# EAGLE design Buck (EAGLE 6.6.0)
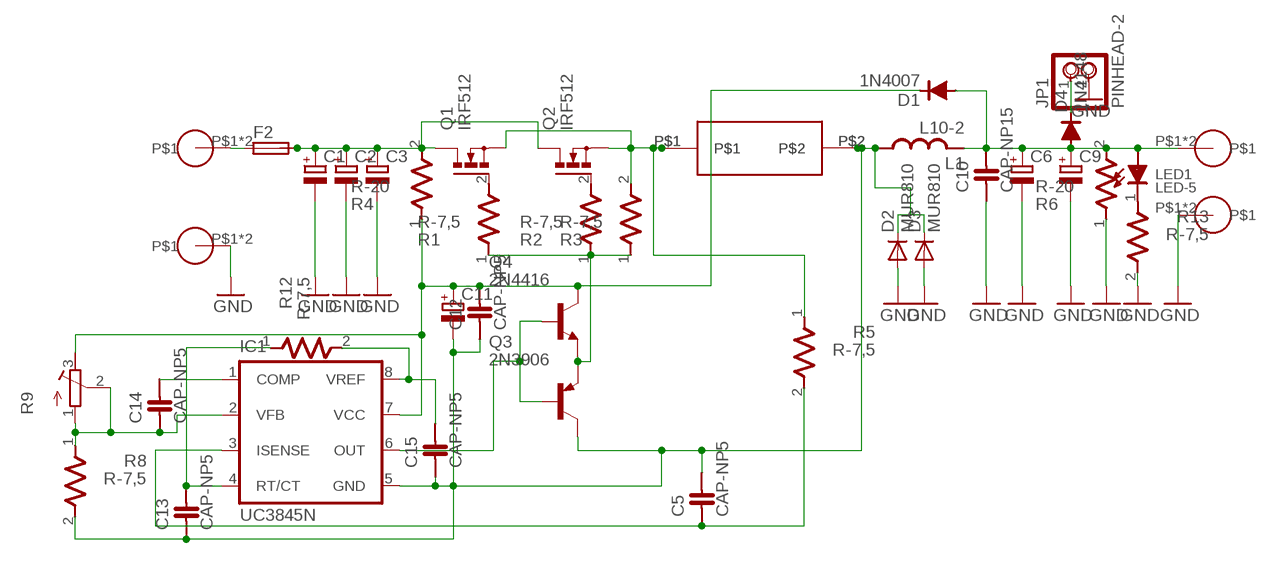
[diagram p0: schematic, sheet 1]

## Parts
C1  CPOL-EUE7.5-18  [E7,5-18]
C2  CPOL-EUE7.5-18  [E7,5-18]
C3  CPOL-EUE7.5-18  [E7,5-18]
C5  CAP-NP5  [CAP-NP5]
C6  CPOL-EUE7.5-18  [E7,5-18]
C9  CPOL-EUE7.5-18  [E7,5-18]
C10  CAP-NP15  [CAP-NP-15]
C11  CPOL-EUE5-8.5  [E5-8,5]
C12  CAP-NP5  [CAP-NP5]
C13  CAP-NP5  [CAP-NP5]
C14  CAP-NP5  [CAP-NP5]
C15  CAP-NP5  [CAP-NP5]
D1  1N4007  [1N4007]
D2  MUR810  [TO220ACS]
D3  MUR810  [TO220ACS]
D4  1N4148  [D-7,5]
F2  LITTLEFUSE  [LITTLEFUSE]
IC1  UC3845N  [DIL08]
JP1  PINHEAD-2  [PINHEAD-2]
L1  L10-2  [L10-2]
LED1  LED-5  [LED5]
Q1  IRF512  [TO220BV]
Q2  IRF512  [TO220BV]
Q3  2N3906  [TO92]
Q4  2N4416  [TO92]
R1  R-7,5  [R-7,5]
R2  R-7,5  [R-7,5]
R3  R-7,5  [R-7,5]
R4  R-20  [R-20]
R5  R-7,5  [R-7,5]
R6  R-20  [R-20]
R8  R-7,5  [R-7,5]
R9  R-TRIMM64W  [RTRIM64W]
R12  R-7,5  [R-7,5]
R13  R-7,5  [R-7,5]
U$1  PIN5MM  [PIN5MM]
U$2  PIN5MM  [PIN5MM]
U$3  SHUNT-0.01R  [SHUNT-0.01R]
U$4  PIN5MM  [PIN5MM]
U$5  PIN5MM  [PIN5MM]
U$6  SHUNT-0.01R  [SHUNT-0.01R]

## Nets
GND: C1.- C2.- C3.- C6.- C9.- C10.1 D2.A D3.A JP1.2 R6.1 R13.2 U$1.P$1 U$1.P$2 U$5.P$1 U$5.P$2
N$1: F2.1 U$2.P$1 U$2.P$2
N$2: C1.+ C2.+ C3.+ F2.2 Q1.D Q2.D R4.2
N$3: Q1.G R1.2
N$4: Q2.G R2.2
N$5: LED1.K R13.1
N$6: D4.C JP1.1
N$7: IC1.6(OUT) Q3.2(B) Q4.2(B)
N$8: Q3.3(E) Q4.3(E) R1.1 R2.1 R3.1
N$9: C5.1 IC1.3(ISENSE) R5.2
N$10: C11.+ C12.2 D1.K IC1.7(VCC) Q4.1(C) R4.1 R9.3(E)
N$11: C6.+ C9.+ C10.2 D1.A D4.A L1.P$3 L1.P$4 LED1.A R6.2 U$4.P$1 U$4.P$2
N$12: C14.2 IC1.1(COMP)
N$13: C5.2 C11.- C12.1 C13.1 C15.1 D2.C D3.C IC1.5(GND) L1.P$1 L1.P$2 Q3.1(C) R8.2 U$3.P$2 U$6.P$2
N$14: Q1.S Q2.S R3.2 R5.1 U$3.P$1 U$6.P$1
N$15: C14.1 IC1.2(VFB) R8.1 R9.1(A) R9.2(S)
N$18: C15.2 IC1.8(VREF) R12.2
N$19: C13.2 IC1.4(RT/CT) R12.1

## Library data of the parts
C1-C3 C6 C9 C11 = LBR inverter true sine:CPOL-EU: POLARIZED CAPACITOR, European symbol
C5 C12-C15 = chuong:CAP-NP5
C10 = chuong:CAP-NP15
D1 = chuong:1N4007
D2 D3 = lbr:MUR810: DIODE
D4 = chuong:1N4148
F2 = LBR inverter true sine:LITTLEFUSE: LITTLEFUSE; OC_FARNELL: unknown; OC_NEWARK: unknown
IC1 = v-reg:UC384*: SMPS Controller Source: http://www.fairchildsemi.com/ds/UC/UC3843.pdf
JP1 = chuong:PINHEAD-2
L1 = lbr:L10-2
LED1 = chuong:LED-5
Q1 Q2 = LBR inverter true sine:IRF512: N-CHANNEL MOS FET
Q3 = lbr:2N3906: PNP Transistor
Q4 = lbr:2N4416: NPN Transistor
R1-R3 R5 R8 R12 R13 = chuong:R-7,5
R4 R6 = chuong:R-20
R9 = chuong:R-TRIMM: Trimm resistor
U$1 U$2 U$4 U$5 = LBR inverter true sine:PIN5MM
U$3 U$6 = Shunt 0.01R:SHUNT-0.01R

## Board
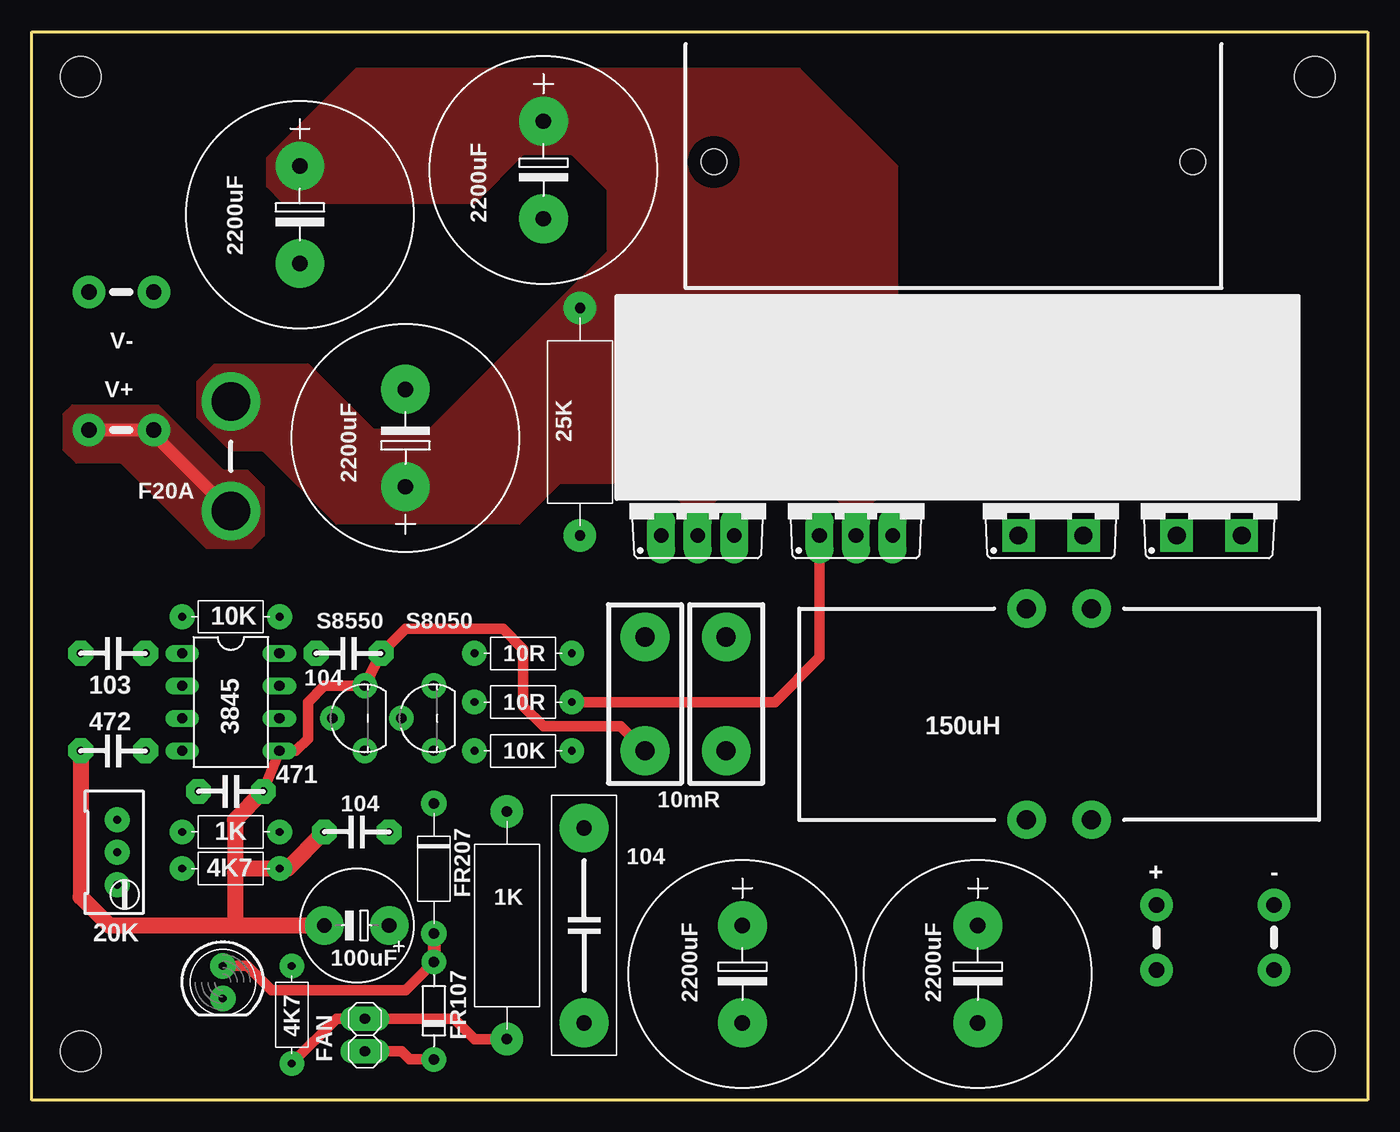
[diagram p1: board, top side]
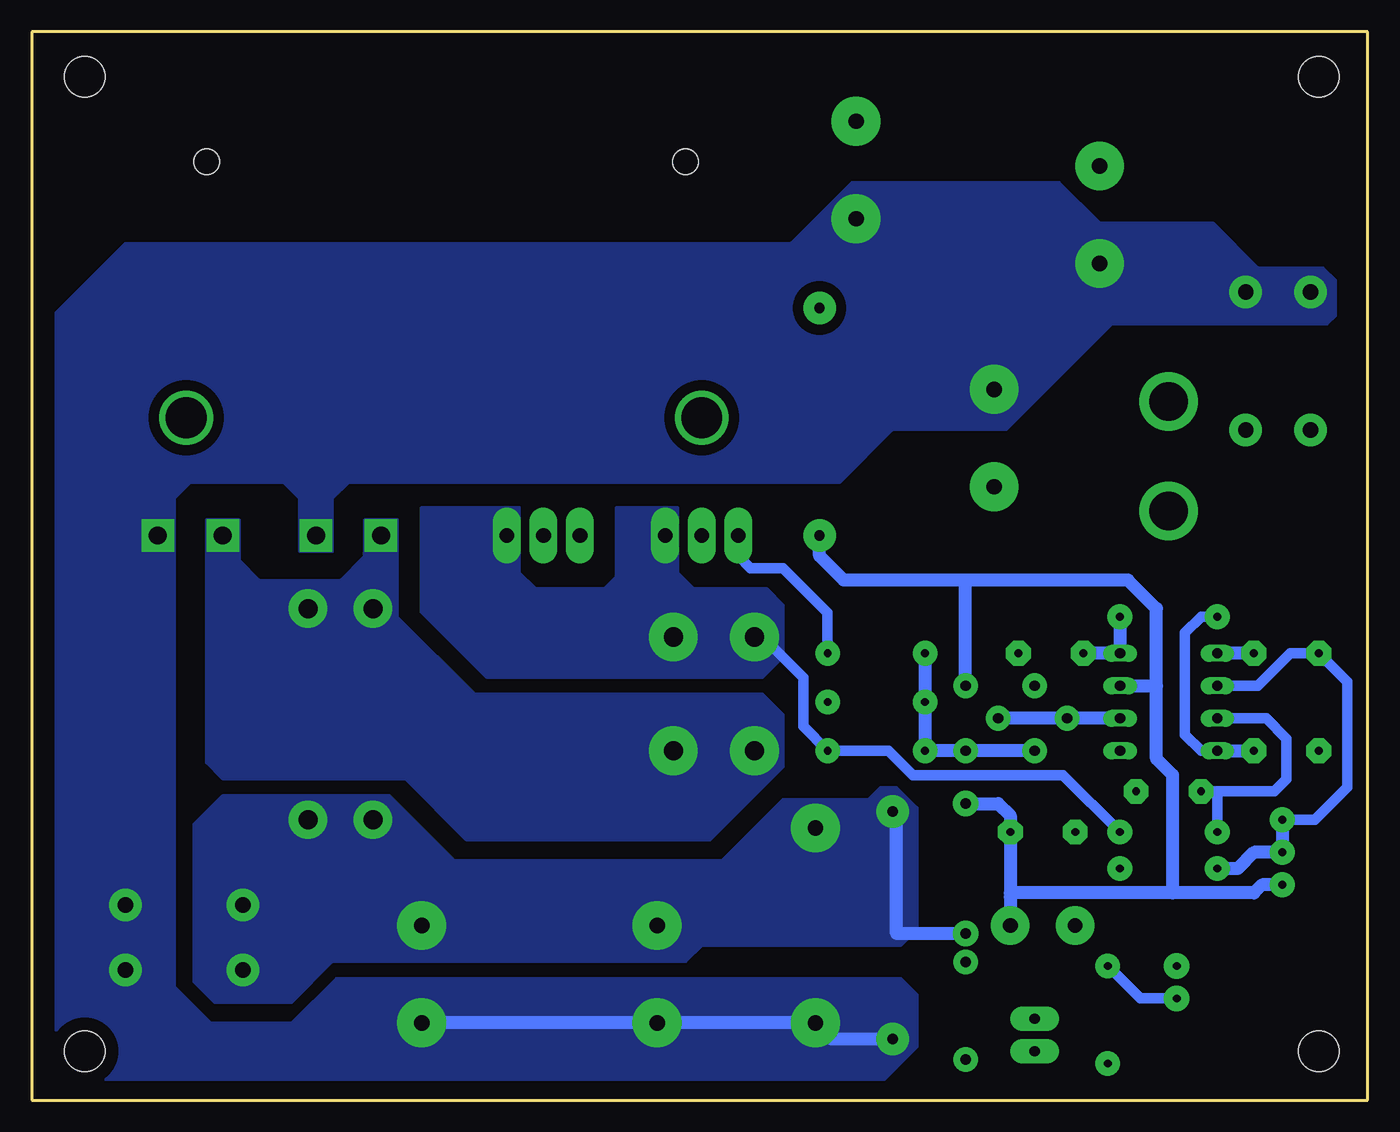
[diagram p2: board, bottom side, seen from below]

Size 104.46 x 83.5 mm. Coordinates in mm from the lower left corner, seen from the top.
Outline: 0,83.5 104.46,83.5 104.46,0 0,0 0,83.5
Copper layers (1*16): Top 0.035mm / dielectric 1.5mm / Bottom 0.035mm
Design rules "default": minimum track width 10mil, minimum drill 24mil, track to track 8mil, track to pad 8mil, pad to pad 8mil, via to via 8mil, smd to smd 8mil, copper to edge 40mil, drill to drill 8mil, minimum pad ring 10mil, minimum via ring 8mil, stop-mask expansion 4mil, vias tented up to drill 0mil, thermal gap 10mil
Holes 2 mm at 90.8,73.34 53.34,73.34
Holes 3.2 mm at 3.81,3.81 100.33,3.81 3.81,80.01 100.33,80.01

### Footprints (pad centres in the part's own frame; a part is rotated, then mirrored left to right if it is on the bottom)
E7,5-18 = drill 1.2 pad 3.81: + -3.81,0; - 3.81,0
CAP-NP5 = drill 0.61 pad 1.93 octagon: 1 -3.81,0; 2 1.27,0
CAP-NP-15 = drill 1.2 pad 3.81: 1 -13.97,0; 2 1.27,0
E5-8,5 = drill 1.15 pad 3: + -2.54,0; - 2.54,0
1N4007 = drill 0.8 pad 2: A 5.08,0; K -5.08,0
TO220ACS = drill 1.4 pad 2.54 square: A 2.54,-2.54; C -2.54,-2.54
D-7,5 = drill 0.8 pad 1.93: A 3.81,0; C -3.81,0
LITTLEFUSE = drill 3 pad 4.572: 1 -5.08,0; 2 3.493,0
DIL08 = drill 0.813 long: 1 -3.81,-3.81; 2 -1.27,-3.81; 3 1.27,-3.81; 4 3.81,-3.81; 5 3.81,3.81; 6 1.27,3.81; 7 -1.27,3.81; 8 -3.81,3.81
PINHEAD-2 = drill 0.813 pad 1.93 long: 1 -1.27,0; 2 1.27,0
L10-2 = drill 1.5 pad 3: P$1 -8.89,2.54; P$2 -8.89,-2.54; P$3 7.62,-2.54; P$4 7.62,2.54
LED5 = drill 0.61 pad 2: A -1.27,0; K 1.27,0
TO220BV = drill 1.15 pad 2.184 long: D 0,-2.54; G -2.857,-2.54; S 2.857,-2.54
TO92 = drill 0.813 pad 1.93: 1 2.54,0; 2 0,2.54; 3 -2.54,0
R-7,5 = drill 0.61 pad 1.93: 1 -3.81,0; 2 3.81,0
R-20 = drill 0.813 pad 2.54: 1 -8.89,0; 2 8.89,0
RTRIM64W = drill 0.61 pad 1.93: 1 0,-2.54; 2 0,0; 3 0,2.54
PIN5MM = drill 1.2 pad 2.54: P$1 -2.54,0; P$2 2.54,0
SHUNT-0.01R = drill 1.5 pad 3.81: P$1 -2.54,-1.27; P$2 6.35,-1.27

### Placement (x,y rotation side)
C1  20.95,69.22 270 top
C2  40.01,72.71 270 top
C3  29.21,51.75 90 top
C5  16.83,24.13 0 top
C6  73.98,9.84 270 top
C9  55.56,9.84 270 top
C10  43.18,20 90 top
C11  25.4,13.65 180 top
C12  26.67,20.96 0 top
C13  7.62,27.3 0 top
C14  7.62,34.92 0 top
C15  23.5,34.92 180 top
D1  31.43,18.1 270 top
D2  79.69,46.67 0 top
D3  92.08,46.67 0 top
D4  31.43,6.99 90 top
F2  15.56,51.12 90 top
IC1  15.56,31.12 270 top
JP1  26.04,5.08 90 top
L1  80.33,29.53 270 top
LED1  14.92,9.21 270 top
Q1  64.45,46.67 0 top
Q2  52.07,46.67 0 top
Q3  26.04,29.85 90 top
Q4  31.43,29.85 90 top
R1  38.42,31.12 0 top
R2  38.42,34.92 0 top
R3  38.42,27.3 0 top
R4  42.86,53.02 90 top
R5  15.56,20.96 180 top
R6  37.15,13.65 90 top
R8  15.56,18.1 0 top
R9  6.67,19.37 180 top
R12  15.56,37.78 0 top
R13  20.32,6.67 270 top
U$1  6.99,63.18 0 top
U$2  6.99,52.39 0 top
U$3  55.56,33.65 270 top
U$4  87.95,12.7 270 top
U$5  97.16,12.7 90 top
U$6  49.21,33.65 270 top

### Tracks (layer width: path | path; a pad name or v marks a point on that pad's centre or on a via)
GND
  Top 0.813: R6.1 34.61,4.76 33.02,6.35 JP1.2 23.81,6.35 R13.2
  Bottom 1.016: R6.1 41.91,4.76 C10.1 C9.- C6.-
  pour Bottom (isolate 0.813, no thermals): 97.16,66.99 45.09,66.99 40.32,71.76 24.13,71.76 20.95,68.58 12.06,68.58 8.57,65.09 3.49,65.09 2.54,64.14 2.54,61.28 3.18,60.64 20,60.64 28.26,52.39 37.15,52.39 41.27,48.26 79.69,48.26 80.96,46.99 80.96,42.86 83.5,42.86 83.5,46.99 84.77,48.26 92.08,48.26 93.34,46.99 93.34,8.89 90.49,6.03 84.14,6.03 80.64,9.52 36.51,9.52 35.24,8.25 35.24,4.13 37.78,1.59 98.74,1.59 102.55,5.4 102.55,61.59
N$1
  Top 1.016: U$2.P$1 U$2.P$2 9.52,52.07 F2.1 15.88,45.72
  pour Top (no thermals): 3.18,54.29 9.84,54.29 14.92,49.21 16.83,49.21 18.1,47.94 18.1,44.13 17.14,43.18 13.65,43.18 6.99,49.85 3.49,49.85 2.54,50.8 2.54,53.66
N$2  (via drill 3.2)
  other vias: 52.07,53.34
  pour Top (isolate 1.016, no thermals): 25.4,80.65 60.01,80.65 67.63,73.03 67.63,48.26 65.41,46.04 65.41,42.86 63.5,42.86 63.5,46.04 61.28,48.26 55.24,48.26 53.02,46.04 53.02,42.86 51.12,42.86 51.12,46.04 48.89,48.26 41.27,48.26 38.1,45.09 23.81,45.09 18.1,50.8 15.56,50.8 13.02,53.34 13.02,56.2 14.29,57.47 21.59,57.47 26.67,52.39 31.12,52.39 45.09,66.36 45.09,71.12 42.23,73.98 38.42,73.98 34.61,70.17 19.68,70.17 18.41,71.44 18.41,73.66
N$3
  Top 0.813: Q1.G 61.59,34.61 58.1,31.12 R1.2
N$4
  Bottom 0.813: R2.2 42.23,38.1 45.72,41.59 48.26,41.59 49.21,42.54 Q2.G
N$5
  Bottom 0.813: LED1.K 17.78,7.94 R13.1
N$6
  Top 0.813: JP1.1 28.89,3.81 29.53,3.18 D4.C
N$7
  Bottom 1.016: IC1.6 Q3.2 Q4.2
N$8
  Bottom 1.016: R2.1 R1.1 34.61,27.94 | 34.61,27.94 R3.1 | Q3.3 Q4.3 33.97,27.3 34.61,27.94
N$9
  Bottom 0.813: IC1.3 7.94,29.85 6.35,28.26 6.35,25.08 7.3,24.13 11.75,24.13 | C5.1 11.75,24.13 | R5.2 11.75,24.13
N$10
  Bottom 1.016: 27.94,16.19 C12.2 27.94,22.23 28.89,23.18 D1.K | 27.94,16.19 27.94,15.87 | 27.94,15.87 C11.+ | R9.3 8.25,16.83 8.89,16.19 15.24,16.19 | 15.24,16.19 27.62,16.19 | 27.62,16.19 27.94,15.87 | 27.94,16.19 27.62,16.19 | 15.24,16.19 15.24,25.4 16.51,26.67 16.51,32.39 | 16.51,32.39 16.51,38.42 18.73,40.64 31.43,40.64 | 31.43,40.64 40.96,40.64 42.86,42.54 R4.1 | IC1.7 16.51,32.39 | Q4.1 31.43,40.64
N$11
  Top 0.813: LED1.A 16.83,10.48 18.73,8.57 29.21,8.57 D4.A
  Top 1.016: D1.A D4.A
  Bottom 1.016: D1.A 36.83,13.02 36.83,22.23 R6.2
  pour Bottom (no thermals): 89.53,23.81 76.52,23.81 71.44,18.73 50.48,18.73 45.72,23.5 39.05,23.5 38.1,24.45 36.83,24.45 35.24,22.86 35.24,13.33 36.51,12.06 52.07,12.06 53.34,10.79 80.96,10.79 84.14,7.62 90.17,7.62 91.76,9.21 91.76,21.59
N$12
  Bottom 1.016: C14.2 IC1.1
N$13
  Top 0.813: U$6.P$2 46.04,29.21 40.01,29.21 38.42,30.8 38.42,35.24 36.83,36.83 29.21,36.83 C15.1 Q3.1 22.86,32.39 21.59,31.12 21.59,28.26 20.64,27.3 IC1.5 C5.2
  Top 1.27: C13.1 3.81,15.87 6.03,13.65 15.88,13.65 | 15.88,13.65 C11.- | C5.2 15.88,21.91 15.88,17.78 | 15.88,17.78 15.88,13.65 | 15.88,17.78 16.19,18.1 R8.2 20,18.1 C12.1
  pour Bottom (no thermals): 69.85,31.75 47.31,31.75 45.72,30.16 45.72,26.04 51.44,20.32 70.48,20.32 75.25,25.08 89.53,25.08 90.8,26.35 90.8,45.4 88.27,45.4 88.27,42.23 86.68,40.64 80.33,40.64 78.42,42.54 78.42,45.4 75.88,45.4 75.88,37.78
N$14
  Bottom 0.813: U$6.P$1 47.63,36.51 44.13,33.02 44.13,29.21 R3.2 37.46,27.3 35.56,25.4 23.81,25.4 R5.1
  pour Bottom (no thermals): 58.74,46.35 53.98,46.35 53.98,41.27 52.7,40 46.99,40 45.72,38.73 45.72,34.61 47.31,33.02 68.9,33.02 73.98,38.1 73.98,46.35 66.36,46.35 66.36,41.27 65.09,40 59.69,40 58.74,40.96
N$15
  Bottom 0.813: R9.1 4.13,21.91 1.59,24.45 1.59,32.7 C14.1 6.03,34.92 8.57,32.39 IC1.2
  Bottom 1.016: R9.1 R9.2 8.89,19.37 10.16,18.1 R8.1
N$16  (via drill 3.2)
  other vias: 92.39,53.34
N$18
  Bottom 1.016: R12.2 IC1.8 C15.2
N$19
  Bottom 0.813: R12.1 13.02,37.78 14.29,36.51 14.29,28.57 13.02,27.3 IC1.4
  Bottom 1.016: IC1.4 C13.2

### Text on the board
tPlace: 2200uF | 2200uF | V- | V+ | 25K | F20A | 2200uF | 10K | S8550 | S8050 | 10R | 104 | 103 | 10R | 472 | 3845 | 150uH | 10K | 471 | 104 | 10mR | FR207 | 1K | 104 | 4K7 | 1K | + | - | 20K | 100uF | FR107 | 4K7 | 2200uF | 2200uF | FAN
